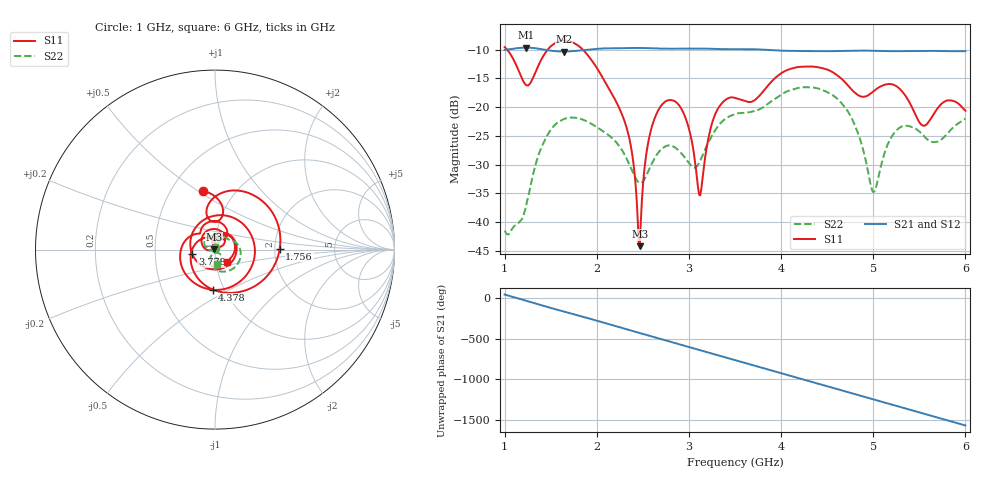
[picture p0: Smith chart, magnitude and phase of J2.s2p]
!Agilent Technologies,E8364B,MY43040528,A.07.50.67
!Agilent E8364B: A.07.50.67
!Date: Sunday, March 01, 2026 18:16:31
!Correction: S11(Full 2 Port(1,2))
!S21(Full 2 Port(1,2))
!S12(Full 2 Port(1,2))
!S22(Full 2 Port(1,2))
!S2P File: Measurements: S11, S21, S12, S22:
# Hz S  dB  R 50
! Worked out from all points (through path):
!   451 points, 1 GHz to 6 GHz, reference 50 ohm
!   highest |S21| = -9.63 dB at 1.233 GHz (marker M1); lowest = -10.3 dB at 1.644 GHz (marker M2)
!   group delay of S21, straight-line fit = 897 ps
!   lowest |S11| = -44.2 dB at 2.467 GHz (marker M3), VSWR 1.01, Z = 49.4 + j0.252 ohm
!   |S11| at or under -10 dB: 1.028 GHz to 1.467 GHz (438.6 MHz wide, 35.2 % of centre); 1.85 GHz to end of sweep
!   |S22| runs from -42.2 to -16.5 dB; largest |S21 - S12| = 0.0015
!   S11 on the Smith chart (normalised r, x): 1 GHz: 0.71, +0.52; 1.756 GHz: 2.13, +0.03; 3.778 GHz: 0.77, -0.04; 4.378 GHz: 0.88, -0.42; 6 GHz: 1.13, -0.15
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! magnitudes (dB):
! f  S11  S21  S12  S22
! 1 GHz  -9.5  -10.0  -10.1  -41.5
! 1.233 GHz  -16.1  -9.6  -9.7  -37.2
! 1.411 GHz  -11.3  -9.9  -10.0  -26.6
! 1.644 GHz  -8.4  -10.3  -10.3  -22.1
! 1.756 GHz  -8.9  -10.2  -10.2  -21.8
! 1.844 GHz  -9.9  -10.1  -10.1  -22.1
! 2.311 GHz  -22.9  -9.7  -9.7  -28.6
! 2.467 GHz  -44.2  -9.7  -9.7  -33.2
! 2.544 GHz  -27.4  -9.7  -9.7  -31.7
! 2.667 GHz  -20.6  -9.8  -9.8  -27.9
! 2.922 GHz  -20.4  -9.8  -9.8  -28.1
! 3.122 GHz  -35.3  -9.8  -9.8  -29.3
! 3.278 GHz  -21.5  -9.9  -9.9  -24.2
! 3.5 GHz  -18.4  -9.9  -9.9  -21.2
! 3.778 GHz  -17.8  -10.0  -10.0  -20.3
! 4.344 GHz  -12.9  -10.2  -10.3  -16.6
! 4.378 GHz  -13.0  -10.2  -10.3  -16.7
! 4.744 GHz  -16.6  -10.2  -10.2  -21.3
! 5 GHz  -17.3  -10.2  -10.2  -34.8
! 5.167 GHz  -16.0  -10.2  -10.3  -26.1
! 5.533 GHz  -23.2  -10.2  -10.2  -24.7
! 6 GHz  -20.6  -10.2  -10.3  -22.0
